ORGANIZATION_BLOCK MAIN:OB1
TITLE=
//COMMENTI DEL PROGRAMMA
//Premere F1 per visualizzare la guida e un esempio di programma
//

BEGIN
NETWORK 1 //Acquisusce segnali analogici
//
//COMMENTI DEL SEGMENTO
//
LD SM0.0
MOVW AIW0 VW0
MOVW AIW2 VW2
MOVW AIW4 VW10

NETWORK 2 //Calcola i Valori di isteresi Sup e inferiore del controllo
//
LD SM0.0
MOVW VW2 VW4
+I VW10 VW4
MOVW VW2 VW6
-I VW10 VW6

NETWORK 3 //Calcola i limiti per il cambio di velocità
//
LD SM0.0
MOVW VW4 VW30
+I +1000 VW30
MOVW VW6 VW32
-I +1000 VW32

NETWORK 4 //Controllo Velocità rotazione motore
//
LDW>= VW0 VW32
AW<= VW0 VW30
MOVW +10000 AQW0
NOT
MOVW +32000 AQW0

NETWORK 5 //Imposta modo Automatico
//
LDN I0.4
= S0.0
R M2.0 2

NETWORK 6 //Imposta modo manuale
//
LD I0.4
= S0.1
R M1.0 2

NETWORK 7 //Inizio segmento manuale
//
LSCR S0.0

NETWORK 8 //Attivazione controllo
//
LD I0.0
O M0.0
A I0.1
AN I0.4
= M0.0
= M3.0

NETWORK 9 //Posizione raggiunta
//
LD M0.0
AW>= VW0 VW6
AW<= VW0 VW4
R M1.0 1
R M1.1 1

NETWORK 10 //Posizione < riferimento
//
LD M0.0
AW< VW0 VW6
R M1.1 1
S M1.0 1

NETWORK 11 //Posizione > Riferimento
//
LD M0.0
AW> VW0 VW4
R M1.0 1
S M1.1 1

NETWORK 12 //Resetta Marker direszione con controllo disabilitato
//
LDN M0.0
R M1.0 2

NETWORK 13 //Fine segmento automatico
//
SCRE

NETWORK 14 //Inizio segmento manuale
//
LSCR S0.1

NETWORK 15
LD I0.2
O I0.3
= M3.1

NETWORK 16
LD I0.2
= M2.0

NETWORK 17
LD I0.3
= M2.1

NETWORK 18 //Fine segmento manuale
//
SCRE

NETWORK 19 //Abilitazione Linea AP
//
LD M3.0
O M3.1
= Q0.2

NETWORK 20 //Abilitazione Marcia Avanti
//
LD M1.0
O M2.0
A I0.6
= Q0.0

NETWORK 21 //Abilitazione marcia Indietro
//
LD M1.1
O M2.1
A I0.5
= Q0.1

NETWORK 22 //Segnalazione posizione raggiunta
//
LDW>= VW0 VW6
AW<= VW0 VW4
LDW<> VW0 VW6
A SM0.5
OLD
LD S0.1
LD S0.0
A M0.0
OLD
ALD
= Q1.0

NETWORK 23 //Segnalazione modo auto attivato
//
LDN I0.4
A M0.0
= Q0.3

NETWORK 24 //Segnalazione fuori corsa destro
//
LDN I0.5
= Q0.4

NETWORK 25 //Segnalazione fuori corsa sinistro
//
LDN I0.6
= Q0.6

END_ORGANIZATION_BLOCK

